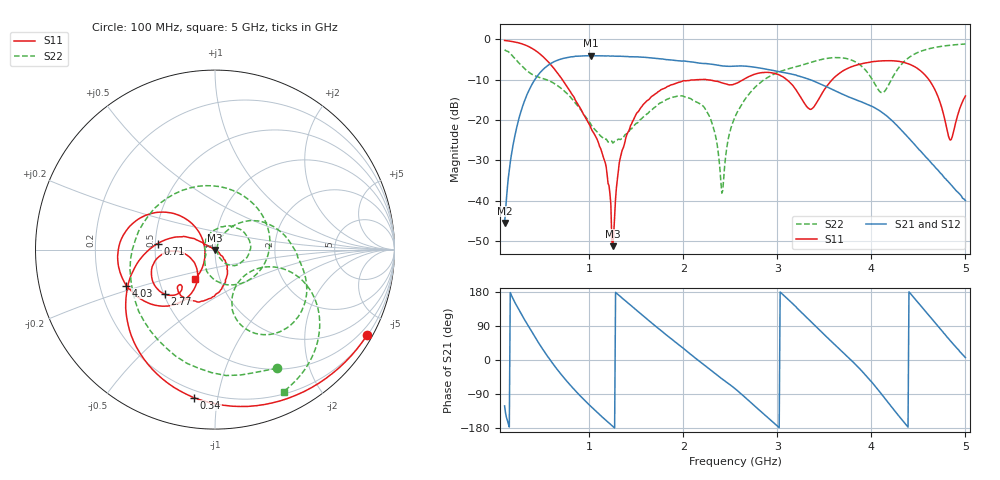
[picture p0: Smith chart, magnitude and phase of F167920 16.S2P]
!  2-Port S-parameters saved by WinCal
! VAR MeasName=S-Parameters (CALIBRATED_DATA) read from VNA (N5242A)
! VAR MeasDate=2016-11-22 9:54:22
! VAR NAME=F167920 16
! VAR FILENAME=F167920 16.S2P
! VAR DATE=2016-11-22 9:54:22
! VAR PHYS_PORTS=1,2
# Hz S DB R 50
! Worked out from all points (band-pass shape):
!   491 points, 100 MHz to 5 GHz, reference 50 ohm
!   highest |S21| = -4.02 dB at 1.02 GHz (marker M1); lowest = -45.5 dB at 100 MHz (marker M2)
!   |S21| within 3 dB of the highest: 529.1 MHz to 2.793 GHz (2.263 GHz wide, 136 % of centre)
!   lowest |S11| = -51.3 dB at 1.25 GHz (marker M3), VSWR 1.01, Z = 50 - j0.27 ohm
!   |S11| at or under -10 dB: 714.8 MHz to 2.131 GHz (1.417 GHz wide, 99.5 % of centre); 3.101 GHz to 3.583 GHz (481.4 MHz wide, 14.4 % of centre); 4.613 GHz to end of sweep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
!   |S22| runs from -38.1 to -1.1 dB; largest |S21 - S12| = 0.0015
!   S11 on the Smith chart (normalised r, x): 100 MHz: 0.22, -3.82; 340 MHz: 0.16, -0.86; 710 MHz: 0.51, +0.04; 2.77 GHz: 0.51, -0.29; 4.03 GHz: 0.32, -0.18; 5 GHz: 0.76, -0.26
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1e8  -0.25 -29.3  -45.51 -121.1  -45.31 -121.8  -2.55 -62.4
2.3e8  -0.74 -66.5  -21.69 142.4  -21.69 142.5  -5.24 -141.1
3.4e8  -1.58 -98.1  -13.56 94.4  -13.57 94.5  -7.78 146.0
5.2e8  -4.51 -146.8  -7.20 23.1  -7.19 23.0  -9.78 32.9
7.1e8  -9.84 174.0  -4.79 -40.7  -4.79 -40.7  -12.29 -49.2
9.2e8  -17.72 151.9  -4.07 -98.5  -4.07 -98.6  -17.74 -110.8
1.02e9  -22.07 150.8  -4.02 -123.2  -4.02 -123.2  -21.17 -130.8
1.17e9  -30.56 153.7  -4.10 -157.6  -4.09 -157.6  -24.77 -153.5
1.25e9  -51.27 -98.3  -4.11 -175.2  -4.10 -175.2  -25.69 -172.6
1.32e9  -30.49 -37.8  -4.16 170.1  -4.15 170.0  -24.75 165.8
1.4e9  -23.64 -44.7  -4.23 153.0  -4.23 153.0  -23.36 141.7
1.74e9  -12.86 -82.2  -4.77 82.3  -4.77 82.3  -15.99 55.4
2.22e9  -9.92 -125.3  -5.98 -12.2  -5.96 -12.3  -16.75 -37.4
2.41e9  -10.75 -135.4  -6.54 -49.5  -6.53 -49.5  -38.12 -10.5
2.55e9  -11.03 -130.8  -6.59 -75.4  -6.58 -75.5  -19.21 59.9
2.77e9  -8.56 -138.4  -6.92 -123.7  -6.90 -123.8  -11.70 38.5
3.37e9  -17.15 -141.2  -10.15 98.1  -10.14 98.1  -5.58 -16.8
4.03e9  -5.47 -157.9  -16.88 -65.9  -16.86 -66.1  -10.75 -70.9
4.19e9  -5.27 -172.1  -19.51 -115.9  -19.51 -116.1  -10.98 -20.6
4.6e9  -9.61 141.3  -29.62 121.3  -29.66 121.2  -2.38 -40.9
4.84e9  -24.96 -176.9  -35.85 50.8  -35.87 50.7  -1.43 -56.2
5e9  -14.03 -124.4  -39.96 6.5  -40.02 6.8  -1.12 -64.3
